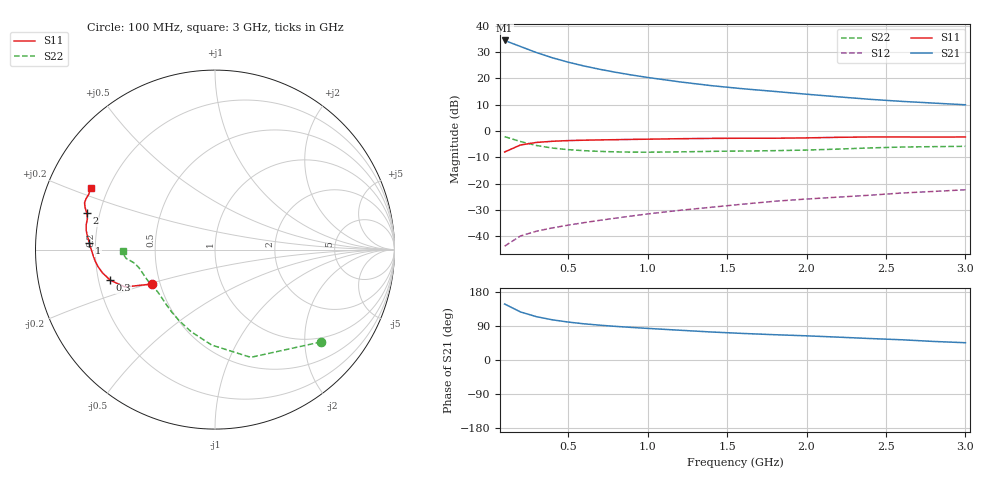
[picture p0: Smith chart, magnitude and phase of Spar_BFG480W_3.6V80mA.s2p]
! Filename: 3_680BFG480.001
! Title: BFG480W
! Bias: Vce=3.6V; Ic=80mA
! Company: NXP Semiconductors NL
! User: Quality&Reliability T&D
! Measure time: 10 Nov 1999 / 12:00:33
#  MHz  S  MA  R 50
! Freq  S11  S21  S12  S22  :
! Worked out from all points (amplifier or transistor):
!   20 points, 100 MHz to 3 GHz, reference 50 ohm
!   highest |S21| = 34.4 dB at 100 MHz (marker M1)
!   |S21| within 3 dB of that: start of sweep to 230.5 MHz
!   unconditionally stable (mu >= 1): 785.8 MHz to end of sweep
!   at 400 MHz: K = 0.76, MSG = 32.3 dB, |S12| = -36.8 dB
!   at 1.2 GHz: K = 1.07, MAG = 22.8 dB, |S12| = -30.1 dB
!   at 3 GHz: K = 1.05, MAG = 14.8 dB, |S12| = -22.3 dB
!   S11 on the Smith chart (normalised r, x): 100 MHz: 0.45, -0.21; 300 MHz: 0.25, -0.13; 1 GHz: 0.18, +0.03; 2 GHz: 0.15, +0.14; 3 GHz: 0.14, +0.23
100  0.4009 -151.4  52.52 147.8  0.006522 69.1  0.7835 -41.0
200  0.5435 -157.5  40.29 126.8  0.0102 59.9  0.6325 -71.6
300  0.6078 -163.7  30.97 114.3  0.01253 57.8  0.5321 -92.0
400  0.6402 -168.3  24.66 106.1  0.01448 59.3  0.476 -106.3
500  0.659 -171.8  20.34 100.2  0.01635 60.9  0.4437 -116.6
600  0.6709 -174.6  17.19 95.5  0.01825 62.9  0.4241 -124.4
700  0.6792 -177.0  14.86 91.8  0.02021 65.0  0.4111 -130.5
800  0.6861 -179.2  13.04 88.7  0.02222 66.7  0.4026 -135.6
900  0.6944 178.8  11.59 86.0  0.0244 68.7  0.398 -140.0
1000  0.701 177.0  10.42 83.4  0.0267 69.8  0.3969 -143.9
1200  0.7155 173.8  8.606 78.6  0.03123 71.7  0.4025 -150.2
1400  0.7258 171.5  7.288 73.9  0.03574 72.8  0.4119 -154.9
1600  0.731 169.1  6.358 70.1  0.04093 73.8  0.4177 -158.5
1800  0.7313 166.5  5.654 66.7  0.04652 74.5  0.4246 -162.3
2000  0.7419 164.2  5.006 63.8  0.05125 75.2  0.4357 -166.7
2200  0.7609 162.0  4.467 60.3  0.0557 75.2  0.4547 -170.4
2400  0.7721 160.3  4.005 56.6  0.06058 74.7  0.4787 -172.8
2600  0.7724 158.6  3.663 53.4  0.06665 74.2  0.4972 -174.3
2800  0.768 156.3  3.396 49.0  0.07138 72.8  0.506 -176.1
3000  0.7727 153.7  3.154 45.6  0.07679 72.1  0.5133 -179.0
